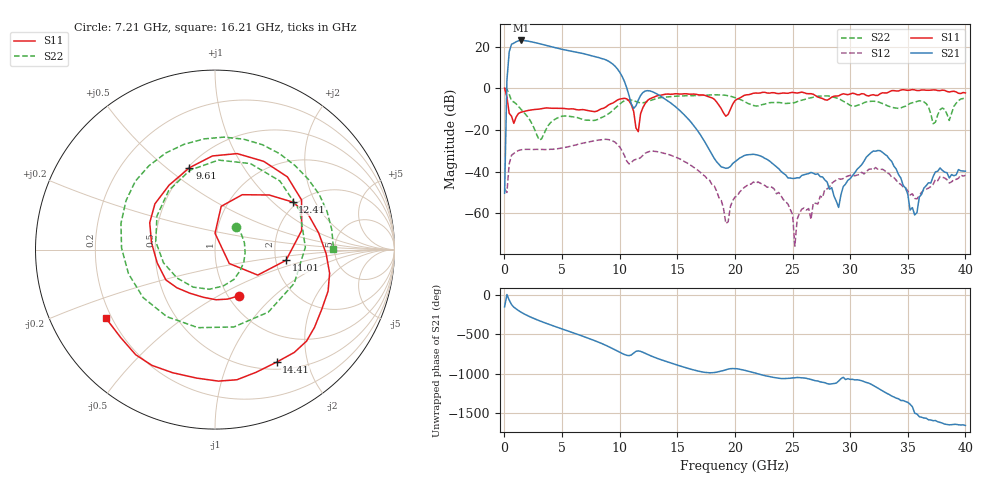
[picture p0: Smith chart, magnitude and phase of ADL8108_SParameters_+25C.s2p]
! Analog Devices, Inc.
! Device:	ADL8108 SN8565
! Description:	"GaAs, pHEMT, MMIC, Low Noise Amplifier, 1.5 GHz to 6 GHz"
! Conditions:	Vdd = 5.0 V
!		Idq = 90 mA
!  Rbias = 1270 Ohm
!		Pin = -25 dBm
!		Operating Temperature = +25 C (at package bottom)
! Board loss de-embedded from S21 magnitude.  All other RF measurements reference to RF coaxial connector.
! Frequency (GHz)	S11_Mag (dB)	S11_Phase (deg)	S21_Mag (dB)	S21_Phase (deg)	S12_Mag (dB)	S12_Phase (deg)	S22_Mag (dB)	S22_Phase (deg)
#  GHZ  S  DB  R 50
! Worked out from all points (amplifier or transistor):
!   201 points, 10 MHz to 40 GHz, reference 50 ohm
!   highest |S21| = 22.9 dB at 1.41 GHz (marker M1)
!   |S21| within 3 dB of that: 545.2 MHz to 4.067 GHz (3.522 GHz wide, 153 % of centre)
!   unconditionally stable (mu >= 1): 57.7 MHz to end of sweep
!   at 6.61 GHz: K = 1.45, MAG = 17.8 dB, |S12| = -26.6 dB
!   at 20 GHz: K = 5758.70, MAG = -32.1 dB, |S12| = -52.2 dB
!   at 40 GHz: K = 1638.86, MAG = -34.2 dB, |S12| = -41.8 dB
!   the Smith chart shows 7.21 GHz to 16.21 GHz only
!   S11 on the Smith chart (normalised r, x): 7.21 GHz: 1.12, -0.63; 9.61 GHz: 0.51, +0.60; 11.01 GHz: 2.28, -0.32; 12.41 GHz: 1.89, +1.35; 14.41 GHz: 0.59, -1.52; 16.21 GHz: 0.18, -0.28
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0.01  -0.01 -5.0  -50.40 -149.4  -48.31 93.3  -0.02 -2.2
0.21  -4.26 -99.9  3.82 6.0  -50.05 -164.7  -0.42 -49.0
0.41  -12.08 -127.8  17.45 -65.0  -36.29 130.9  -2.93 -94.8
0.61  -13.45 -143.1  21.09 -121.2  -32.18 79.5  -6.01 -117.6
1.01  -13.84 -137.4  22.27 -176.2  -30.56 36.4  -7.51 -162.4
1.41  -11.57 -162.5  22.91 144.3  -29.60 8.5  -9.98 158.3
2.21  -10.54 161.7  22.41 84.0  -29.36 -29.6  -15.34 95.5
3.41  -9.59 118.4  20.82 12.2  -29.44 -69.3  -22.11 -72.6
5.01  -9.67 56.7  18.65 -70.7  -28.70 -112.5  -13.44 -171.7
6.81  -10.26 -39.2  16.64 -163.4  -26.38 -169.6  -15.06 81.0
7.21  -10.76 -62.7  16.09 174.8  -25.93 175.2  -15.32 47.1
8.41  -9.85 -148.3  14.25 106.9  -24.77 123.9  -14.11 -57.6
9.61  -6.42 107.4  10.47 23.2  -25.97 54.1  -9.55 172.3
11.01  -7.96 -8.6  -7.57 -40.4  -35.64 38.4  -5.68 24.7
12.41  -5.90 31.5  -1.18 -33.3  -30.66 8.5  -6.35 -146.2
13.41  -3.46 -20.2  -3.34 -92.0  -30.59 -40.0  -4.66 139.4
14.41  -2.92 -61.3  -7.01 -140.8  -32.11 -82.8  -4.03 85.4
16.21  -2.88 -147.8  -16.47 137.6  -37.16 -158.7  -3.61 0.3
20.2  -5.23 153.8  -34.36 144.8  -51.80 -157.2  -4.87 -174.9
26.8  -2.91 -89.4  -40.84 0.3  -55.07 111.8  -4.35 109.0
33.4  -1.71 102.9  -33.98 177.3  -41.12 -128.1  -8.77 118.6
40  -2.28 -17.6  -39.84 145.5  -41.84 131.2  -4.71 -43.0
